(* Logix 5000 AddOnInstructionDefinition export; software revision 16.04 *)

TYPE AKD_Status :   // All connections to the drive ethernet module are established and data is successfully transferring.
STRUCT
   Profile_In_Progress : BOOL;   // Profile Move In Progress
   Block_In_Execution : BOOL;   // Block In Execution
   On_Target_Position : BOOL;   // On Target Position (1=Current Position Equals Last Target Position)
   General_Fault : BOOL;   // General Fault
   Current_Direction : BOOL;   // Current Motor Direction (0=Reverse, 1=Forward)
   Home_Level : BOOL;   // Level of Home Input
   Reg_Level : BOOL;   // Level of Registration Input
   Enable : BOOL;   // State of Enable Output
   Fault_Input_Fault : BOOL;   // Fault Input Active
   Fwd_Limit : BOOL;   // Forward Input Active
   Rev_Limit : BOOL;   // Reverse Input Active
   Positive_Limit : BOOL;   // Positive Software Limit Exceeded
   Negative_Limit : BOOL;   // Negative Software Limit Exceeded
   FE_Fault : BOOL;   // Following Error Fault
   Block_Fault : BOOL;   // Block Execution Fault
   Load_Complete : BOOL;   // Command Message Successfully Loaded
END_STRUCT
END_TYPE

TYPE AKD_Axis :   // Axis Data:
STRUCT
   Control : AKD_Control;   // Control bits to send to the drive
   Status : AKD_Status;   // Status bits received from the drive
   Input : AB:ETHERNET_MODULE_SINT_64Bytes:I:0;   // Data from the drive
   Output : AB:ETHERNET_MODULE_SINT_64Bytes:O:0;   // Data to the drive
   ResponseMsgType : SINT;   // Response type contained in latest IO response from drive. Used to check for errors
   CommandTimeout : INT;   // Time to allow for command response from drive. Dependent on scan rate and communicaiton rate
   PositionFeedback : DINT;   // Actual Position Value
   VelocityFeedback : DINT;   // Actual Velocity Value
END_STRUCT
END_TYPE

TYPE AKD_Control :   // Send Explicit Message
STRUCT
   Load_Data_Start_Profile : BOOL;   // Load Command Data / Start Profile Move
   Start_Block : BOOL;   // Execute Command block or block chain
   Incremental : BOOL;   // Incremental Position (0=Absolute, 1=Incremental)
   Direction : BOOL;   // Direction in Velocity Mode (0=Reverse, 1=Forward)
   Smooth_Stop : BOOL;   // Smooth / Controlled Stop w/ Deceleration
   Hard_Stop : BOOL;   // Hard / Immediate Stop
   Reg_Arm : BOOL;   // Arm the Registration Input
   Enable : BOOL;   // Enable Output
END_STRUCT
END_TYPE

ADD_ON_INSTRUCTION AKD_Enable   (* revision 2.0, ExecutePrescan, ExecuteEnableInFalse *)
// Enables Drive
VAR_OUTPUT
   DN : BOOL; {visible}   // Command Successful
   ER : BOOL; {visible}   // Error
END_VAR
VAR_IN_OUT
   Axis : AKD_Axis; {required}
END_VAR
VAR
   Command_Timeout : TIMER;   // Timeout Timer
   Transition : BOOL;   // Marker to transition enable bit if required.
   Transition_Complete : BOOL;   // Flag to indicate that no further transistion is required.
END_VAR

ROUTINE EnableInFalse   (* ladder *)
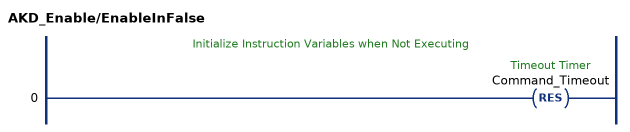
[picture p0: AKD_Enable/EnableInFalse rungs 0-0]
   // Initialize Instruction Variables when Not Executing
   0: RES(Command_Timeout);
END_ROUTINE

ROUTINE Logic   (* ladder *)
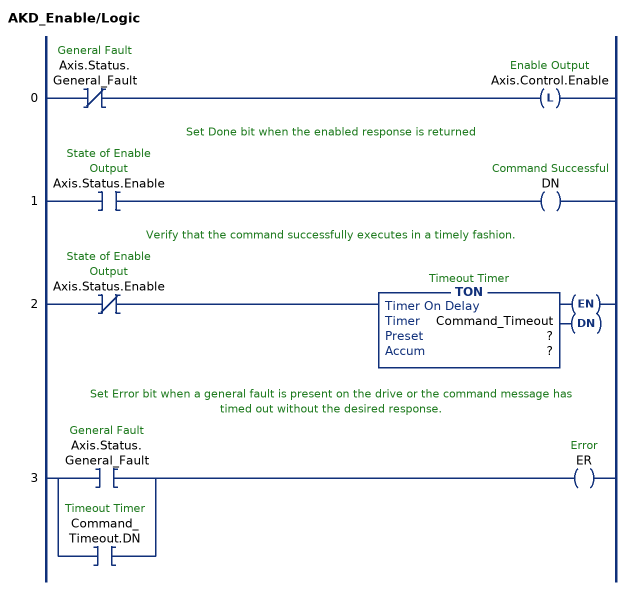
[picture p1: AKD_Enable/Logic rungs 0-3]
   0: XIO(Axis.Status.General_Fault)OTL(Axis.Control.Enable);
   // Set Done bit when the enabled response is returned
   1: XIC(Axis.Status.Enable)OTE(DN);
   // Verify that the command successfully executes in a timely fashion.
   2: XIO(Axis.Status.Enable)TON(Command_Timeout,?,?);
   // Set Error bit when a general fault is present on the drive or the command message has timed out without the desired response.
   3: [XIC(Axis.Status.General_Fault) ,XIC(Command_Timeout.DN) ]OTE(ER);
END_ROUTINE

ROUTINE Prescan   (* ladder *)
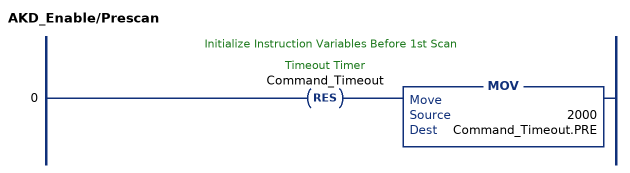
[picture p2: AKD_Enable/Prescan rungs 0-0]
   // Initialize Instruction Variables Before 1st Scan
   0: RES(Command_Timeout)MOV(2000,Command_Timeout.PRE);
END_ROUTINE
END_ADD_ON_INSTRUCTION
